TYPE "ST_AcyclicWriteRequest"
VERSION : 0.1


  STRUCT
   byServiceID : BYTE ;	//Service ID |  0x11 = Write object acyclic
   dwMessageID : DWORD ;	//Message ID | Free usable message ID of the application | Can be set from the cl
   dwDataLength : DWORD ;	//Data length | 0x04 (Object index, Sub index, Data type) + data length of the Ob
   byAcknowledge : BYTE ;	//Acknowledge | Can be set to 0x00 in this request
   dwWriteType : DWORD ;	//Write type | 0x00 = Single write object | Write object with one sub index (e.g.
   wIndex : WORD ;	//Index | Index of the object to be written
   bySubIndex : BYTE ;	//Sub Index | Sub Index of the object to be written
   byDataType : BYTE ;	//Data type | Data type of the object to be written
   abyDataByte : ARRAY  [1 .. 76 ] OF //Data bytes | Data bytes of the value to be written
   BYTE ;
  END_STRUCT ;
END_TYPE

